(* Logix 5000 DataType export Banner_IO_Metrics_v4; software revision 33.00 *)

TYPE Banner_IO_Metrics_v4 :
STRUCT
   Port_1_DI1_Count : DINT;
   Port_1_DI1_Duration : DINT;
   Port_1_DI1_Events_per_Minute : DINT;
   Port_1_DI1_Counts_per_Minute : DINT;
   Port_1_DI1_Totalizer_Counter : DINT;
   Port_1_DI2_Count : DINT;
   Port_1_DI2_Duration : DINT;
   Port_1_DI2_Events_per_Minute : DINT;
   Port_1_DI2_Counts_per_Minute : DINT;
   Port_1_DI2_Totalizer_Counter : DINT;
END_STRUCT
END_TYPE
